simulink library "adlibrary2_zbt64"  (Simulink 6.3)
undefined symbols (not defined in the file or in its folder): Bit, blackbox2, blue, gcbh, Inactive, Location, Lower, VER_STRING_GOES_HERE, white, Width, xlBlockLoadCallback, zbt64_config
libraries: xbsIndex_r4 x21, adlibrary2_zbt64 x1

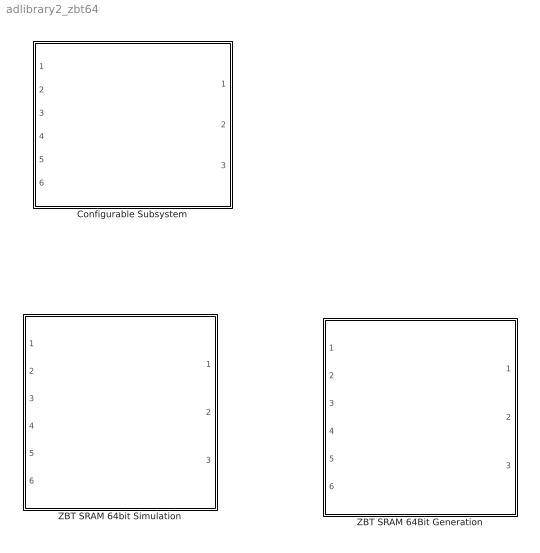
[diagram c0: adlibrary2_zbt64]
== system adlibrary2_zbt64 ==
  Configurable Subsystem : Subsystem  Tag=configX  BlockChoice=ZBT SRAM 64bit Simulation
  ZBT SRAM 64Bit Generation : Subsystem
  ZBT SRAM 64bit Simulation : Subsystem

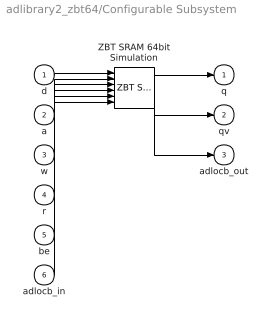
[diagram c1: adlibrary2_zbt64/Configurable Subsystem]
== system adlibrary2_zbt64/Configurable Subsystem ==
  d : Inport
  a : Inport  Port=2
  w : Inport  Port=3
  r : Inport  Port=4
  be : Inport  Port=5
  adlocb_in : Inport  Port=6
  ZBT SRAM 64bit Simulation : adlibrary2_zbt64/ZBT SRAM 64bit Simulation
  q : Outport
  qv : Outport  Port=2
  adlocb_out : Outport  Port=3
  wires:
  d/1 -> ZBT SRAM 64bit Simulation/1
  a/1 -> ZBT SRAM 64bit Simulation/2
  w/1 -> ZBT SRAM 64bit Simulation/3
  r/1 -> ZBT SRAM 64bit Simulation/4
  be/1 -> ZBT SRAM 64bit Simulation/5
  adlocb_in/1 -> ZBT SRAM 64bit Simulation/6
  ZBT SRAM 64bit Simulation/1 -> q/1
  ZBT SRAM 64bit Simulation/2 -> qv/1
  ZBT SRAM 64bit Simulation/3 -> adlocb_out/1

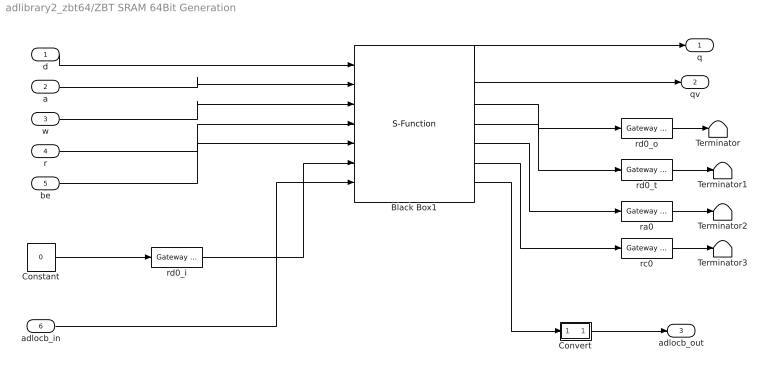
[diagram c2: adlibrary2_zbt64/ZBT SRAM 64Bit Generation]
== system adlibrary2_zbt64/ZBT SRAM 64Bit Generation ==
  d : Inport
  a : Inport  Port=2
  w : Inport  Port=3
  r : Inport  Port=4
  be : Inport  Port=5
  adlocb_in : Inport  Port=6
  Black Box1 : S-Function  LoadFcn=xlBlockLoadCallback(gcbh);  FunctionName=sysgen  Parameters=ptable_  mask(Xilinx Black Box Block){infoedit=Incorporates black box HDL and simulation model into a System Generator design.<P><P>You must supply a Black Box with certain information about the HDL component you would like to bring into System Generator. This information is provided through a Matlab function.<P><P>When "Simulation mode" is set to "Inactive", you will typically want to provide a separate simulation model by using a Simulation 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, init_code=zbt64_config, sim_method=Inactive, sim_method_sgadvanced=, engine_block=, xl_use_area=off, xl_use_area_sgadvanced=, xl_area=[0,0,0,0,0,0,0], block_version=VER_STRING_GOES_HERE, has_advanced_control=0, sggui_pos=20,20,356,367, block_type=blackbox2, sg_icon_stat=130,170,7,7,white,blue,0,1b6b346b, sg_mask_display=fprintf('','COMMENT: begin icon graphics '); patch([0 130 130 0 ],[0 0 170 170 ],[0.77 0.82 0.91]); patch([31 9 39 9 31 65 74 83 120 91 63 43 74 43 63 91 120 83 74 65 31 ],[34 56 86 116 138 138 129 138 138 109 137 117 86 55 35 63 34 34 43 34 34 ],[0.98 0.96 0.92]); plot([0 0 130 130 0 ],[0 170 170 0 0 ]); fprintf('','COMMENT: end icon graphics');  fprintf('','COMMENT: begin icon text '); color('bl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, sg_list_contents=, adlocb_devid=0}
      mask prompts: infoedit ""; init_code "Block configuration m-function"; sim_method "Simulation mode"; engine_block "HDL co-simulator to use  (specify helper block by name)"; xl_use_area "Define FPGA area for resource estimation"; xl_area "FPGA area [slices, FFs, BRAMs, LUTs, IOBs, emb. mults, TBUFs]"; block_version ""; has_advanced_control ""; sggui_pos ""; block_type ""; sg_icon_stat ""; sg_mask_display ""; sg_list_contents ""; adlocb_devid "ADLOCB DEV ID"
      mask help: Incorporates black box HDL and simulation model into a System Generator design. You must supply a Black Box with certain information about the HDL component you would like to bring into System Generator. This information is provided through a Matlab function. When "Simulation mode" is set to "Inactive", you will typically want to provide a separate simulation model by using a Simulation Multiplexer. When "Simulation mode" is set to "External co-simulator", you must include a ModelSim block in the design.
      mask init:
      | xlMungeMaskParams;
      | 
      | mdlPath = xlGetMdlDir(bdroot);
      | 
      | refBlk = get_param(gcb,'referenceBlock');
      | if (isempty(refBlk) | strncmp(refBlk,'xbsIndex',8))
      | srcPath = mdlPath;
      | else
      | srcPath = xlPathToReference;
      | if (isempty(srcPath))
      | srcPath = mdlPath;
      | end
      | end
      | 
      | if (sim_method==3)
      | validEngineBlock = 0;
      | try
      | engineBlock = xlBlockNameRelPath(get_param(gcb,'Parent'),engine_block);
      | catch
      | engineBlock = '//';
      | end
      | try 
      | engineWorkDir = get_param(engineBlock,'dir');
      | validEngineBlock = 1;
      | engine_handle = get_param(engineBlock,'Handle');
      | catch
      | end
      | end
      | 
      | % build black box config function
      | block_config = ['sysgen:black_box_config:' init_code];
      | 
      | serialized_declarations = '{''engine_handle''=>''Double'',''sim_method''=>''Int'',''validEngineBlock''=>''Int'',''engineWorkDir''=>''String'',''engine_block''=>''String'',''init_code''=>''String'',''mdlPath''=>''String'',''srcPath''=>''String'',''block_config''=>''String'',}';
      | ptable_ = xlblockprep(get_param(gcb, 'MaskWSVariables'));
  Constant : Constant  Value=0
  Convert : Subsystem
  Terminator{,1..3} (4 alike) : Terminator
  ra0 : xbsIndex_r4/Gateway Out  hdl_port=on  timing_constraint=None  locs_specified=off  LOCs={}  block_type=gatewayout
  rc0 : xbsIndex_r4/Gateway Out  hdl_port=on  timing_constraint=None  locs_specified=off  LOCs={}  block_type=gatewayout
  rd0_i : xbsIndex_r4/Gateway In  arith_type=Unsigned  n_bits=64  bin_pt=0  period=ad_get_simulink_period  dbl_ovrd=off  timing_constraint=None  locs_specified=off  LOCs={}  block_type=gatewayin
  rd0_o : xbsIndex_r4/Gateway Out  hdl_port=on  timing_constraint=None  locs_specified=off  LOCs={}  block_type=gatewayout
  rd0_t : xbsIndex_r4/Gateway Out  hdl_port=on  timing_constraint=None  locs_specified=off  LOCs={}  block_type=gatewayout
  q : Outport
  qv : Outport  Port=2
  adlocb_out : Outport  Port=3
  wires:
  Convert/1(out0) -> adlocb_out/1
  Black Box1/7 -> Convert/1(in0)
  adlocb_in/1 -> Black Box1/7
  Black Box1/6 -> rc0/1
  Black Box1/5 -> ra0/1
  Black Box1/4 -> rd0_t/1
  Black Box1/3 -> rd0_o/1
  Black Box1/2 -> qv/1
  be/1 -> Black Box1/5
  r/1 -> Black Box1/4
  w/1 -> Black Box1/3
  a/1 -> Black Box1/2
  rc0/1 -> Terminator3/1
  ra0/1 -> Terminator2/1
  rd0_t/1 -> Terminator1/1
  rd0_o/1 -> Terminator/1
  Constant/1 -> rd0_i/1
  rd0_i/1 -> Black Box1/6
  Black Box1/1 -> q/1
  d/1 -> Black Box1/1

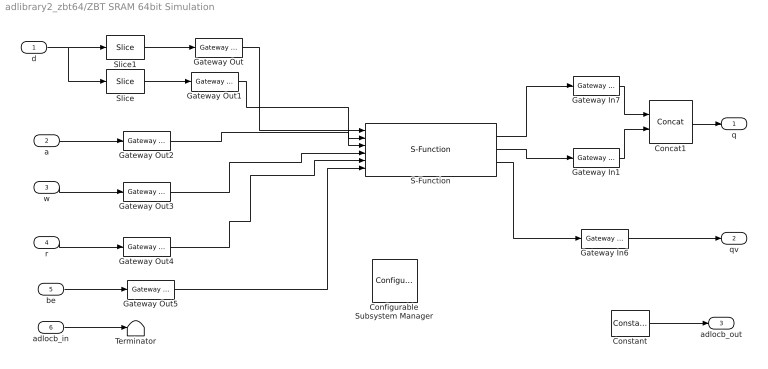
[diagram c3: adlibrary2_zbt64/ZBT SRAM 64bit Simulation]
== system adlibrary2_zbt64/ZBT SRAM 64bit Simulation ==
  d : Inport
  a : Inport  Port=2
  w : Inport  Port=3
  r : Inport  Port=4
  be : Inport  Port=5
  adlocb_in : Inport  Port=6
  Concat1 : xbsIndex_r4/Concat  num_inputs=2  dbl_ovrd=off  block_type=concat
  Configurable Subsystem Manager : xbsIndex_r4/Configurable Subsystem Manager  Tag=xcfgMgr  block_type=configsubsys
  Constant : xbsIndex_r4/Constant  arith_type=Unsigned  const=0  n_bits=66  bin_pt=0  explicit_period=on  period=ad_get_simulink_period  equ=P=C  opselect=C  inp2=PCIN>>17  opr=+  inp1=P  carry=CIN  dbl_ovrd=off  block_type=constant
  Gateway In1 : xbsIndex_r4/Gateway In  arith_type=Unsigned  n_bits=32  bin_pt=0  period=ad_get_simulink_period  dbl_ovrd=on  timing_constraint=None  locs_specified=off  LOCs={}  block_type=gatewayin
  Gateway In6 : xbsIndex_r4/Gateway In  arith_type=Boolean  n_bits=1  bin_pt=0  period=ad_get_simulink_period  dbl_ovrd=on  timing_constraint=None  locs_specified=off  LOCs={}  block_type=gatewayin
  Gateway In7 : xbsIndex_r4/Gateway In  arith_type=Unsigned  n_bits=32  bin_pt=0  period=ad_get_simulink_period  dbl_ovrd=on  timing_constraint=None  locs_specified=off  LOCs={}  block_type=gatewayin
  Gateway Out{,1..5} (6 alike) : xbsIndex_r4/Gateway Out  hdl_port=off  timing_constraint=None  locs_specified=off  LOCs={}  block_type=gatewayout
  S-Function : S-Function  FunctionName=zbt64  Parameters=0
  Slice : xbsIndex_r4/Slice  nbits=32  boolean_output=off  mode=Lower Bit Location + Width  bit1=0  base1=MSB of Input  bit0=0  base0=LSB of Input  dbl_ovrd=off  block_type=slice
  Slice1 : xbsIndex_r4/Slice  nbits=32  boolean_output=off  mode=Lower Bit Location + Width  bit1=0  base1=MSB of Input  bit0=32  base0=LSB of Input  dbl_ovrd=off  block_type=slice
  Terminator : Terminator
  q : Outport
  qv : Outport  Port=2
  adlocb_out : Outport  Port=3
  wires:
  Concat1/1 -> q/1
  Gateway In1/1 -> Concat1/2
  Gateway In7/1 -> Concat1/1
  d/1 -> Slice/1, Slice1/1
  Slice/1 -> Gateway Out1/1
  Slice1/1 -> Gateway Out/1
  Gateway Out5/1 -> S-Function/6
  be/1 -> Gateway Out5/1
  S-Function/3 -> Gateway In6/1
  Gateway In6/1 -> qv/1
  S-Function/2 -> Gateway In1/1
  Gateway Out4/1 -> S-Function/5
  r/1 -> Gateway Out4/1
  Gateway Out3/1 -> S-Function/4
  Gateway Out2/1 -> S-Function/3
  Gateway Out1/1 -> S-Function/2
  Gateway Out/1 -> S-Function/1
  S-Function/1 -> Gateway In7/1
  w/1 -> Gateway Out3/1
  a/1 -> Gateway Out2/1
  Constant/1 -> adlocb_out/1
  adlocb_in/1 -> Terminator/1

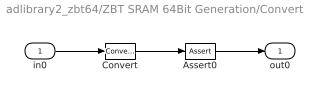
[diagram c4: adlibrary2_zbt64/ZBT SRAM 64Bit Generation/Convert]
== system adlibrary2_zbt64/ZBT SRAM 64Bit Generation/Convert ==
  in0 : Inport
  Assert0 : xbsIndex_r4/Assert  assert_type=off  type_source=Explicitly  arith_type="Signed  (2's comp)"  n_bits=16  bin_pt=14  assert_rate=on  rate_source=Explicitly  period=ad_get_simulink_period  output_port=on  block_type=assert
  Convert : xbsIndex_r4/Convert  arith_type=Unsigned  n_bits=66  bin_pt=0  quantization=Truncate  overflow=Wrap  latency=0  dbl_ovrd=off  pipeline=off  block_type=convert
  out0 : Outport
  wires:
  Assert0/1 -> out0/1
  Convert/1 -> Assert0/1
  in0/1 -> Convert/1
